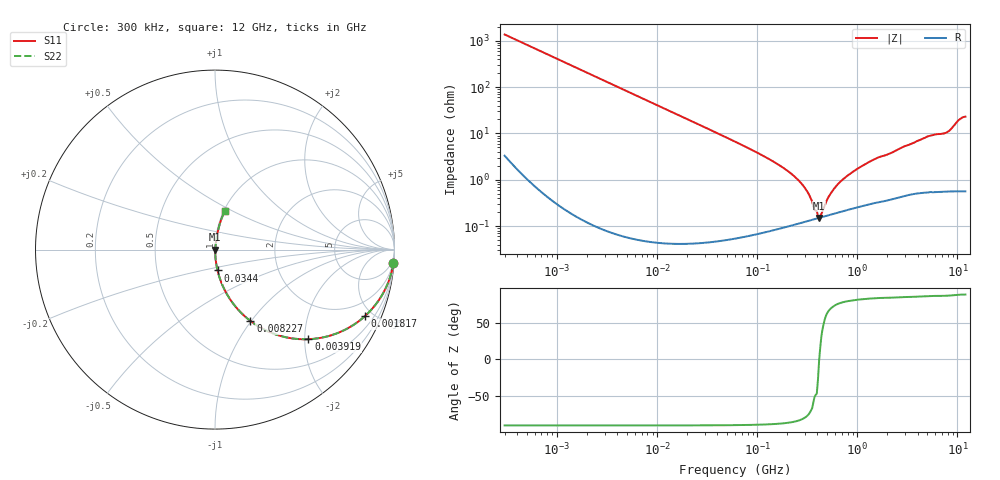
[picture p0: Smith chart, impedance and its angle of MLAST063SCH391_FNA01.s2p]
! MLAST063SCH391_FNA01  S-PARAMETER MODEL  ( General Type )
! Model Generated by TAIYO YUDEN Corporation (http://www.ty-top.com)
! Version 1.0
! TAIYO YUDEN Control No. 160830
! Copyright(c) 2016 TAIYO YUDEN CO.,LTD. All Rights Reserved.
! Product Description (link to TY-COMPAS)
! https://ds.yuden.co.jp/TYCOMPAS/or/detail?pn=MLAST063SCH391JFNA01&u=M
! Products Name : Multilayer Ceramic Capacitors
! Characteristics :
!  Capacitance : 390 pF , Rated Voltage : 25V , TCC : CH / C0H
!  Case Size : 0.6 x 0.3 / 0.024 x 0.012 [mm/inch] , Thickness : 0.3 / 0.012 [mm/inch]
!  (Conditions: Temperature = 25 degC , DC Bias Current/Voltage = 0A / 0V)
! External Node Assignments :
!  1  o---| |---o  2
! GND o---------o GND
! Frequency Range : 0.3MHz  -  12000MHz  [ 401 STEP ]
# MHz S RI R 50
! Freq[MHz].  S11 Real  S11 Imag  S21 Real  S21 Imag  S12 Real  S12 Imag  S22 Real  S22 Imag
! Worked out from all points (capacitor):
!   401 points, 300 kHz to 12 GHz, reference 50 ohm
!   read as one part in series: C = 390 pF near 316.3 kHz
!   lowest |Z| = 151 mohm at 415 MHz (marker M1)
!   series resonance near 416.1 MHz, so ESL is about 380 pH
!   S11 on the Smith chart (normalised r, x): 300 kHz: 1, -27; 1.817 MHz: 1.00, -4.49; 3.919 MHz: 1.00, -2.08; 8.227 MHz: 1.00, -0.99; 34.4 MHz: 1.00, -0.24; 12 GHz: 1.01, +0.46
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0.3  0.9944 -0.0731  0.00555 0.0731  0.00555 0.0731  0.9944 -0.0731
0.888858  0.9546 -0.2079  0.0454 0.2079  0.0454 0.2079  0.9546 -0.2079
1.769972  0.8415 -0.3649  0.1585 0.3649  0.1585 0.3649  0.8415 -0.3649
1.817488  0.8343 -0.3715  0.1657 0.3715  0.1657 0.3715  0.8343 -0.3715
3.918509  0.5202 -0.4993  0.4798 0.4993  0.4798 0.4993  0.5202 -0.4993
8.227445  0.1975 -0.3977  0.8025 0.3977  0.8025 0.3977  0.1975 -0.3977
10.44266  0.1326 -0.3386  0.8674 0.3386  0.8674 0.3386  0.1326 -0.3386
34.39878  0.0141 -0.1161  0.9859 0.1161  0.9859 0.1161  0.0141 -0.1161
60  0.00495 -0.0662  0.9951 0.0662  0.9951 0.0662  0.00495 -0.0662
213.9924  0.00121 -0.014  0.9988 0.014  0.9988 0.014  0.00121 -0.014
294.0765  0.00127 -0.00692  0.9987 0.00692  0.9987 0.00692  0.00127 -0.00692
353.9943  0.00138 -0.00313  0.9986 0.00313  0.9986 0.00313  0.00138 -0.00313
393.5654  0.00146 -0.00154  0.9985 0.00154  0.9985 0.00154  0.00146 -0.00154
414.98  0.00151 -4.84e-05  0.9985 4.84e-05  0.9985 4.84e-05  0.00151 -4.84e-05
437.5599  0.00156 0.000963  0.9984 -0.000963  0.9984 -0.000963  0.00156 0.000963
555.3718  0.00182 0.00515  0.9982 -0.00515  0.9982 -0.00515  0.00182 0.00515
723.8279  0.00221 0.0101  0.9978 -0.0101  0.9978 -0.0101  0.00221 0.0101
1229.528  0.00334 0.0222  0.9967 -0.0222  0.9967 -0.0222  0.00334 0.0222
2088.533  0.00496 0.036  0.995 -0.036  0.995 -0.036  0.00496 0.036
5006.236  0.0125 0.0842  0.9875 -0.0842  0.9875 -0.0842  0.0125 0.0842
7648.807  0.0158 0.1006  0.9842 -0.1006  0.9842 -0.1006  0.0158 0.1006
12000  0.055 0.216  0.945 -0.216  0.945 -0.216  0.055 0.216
